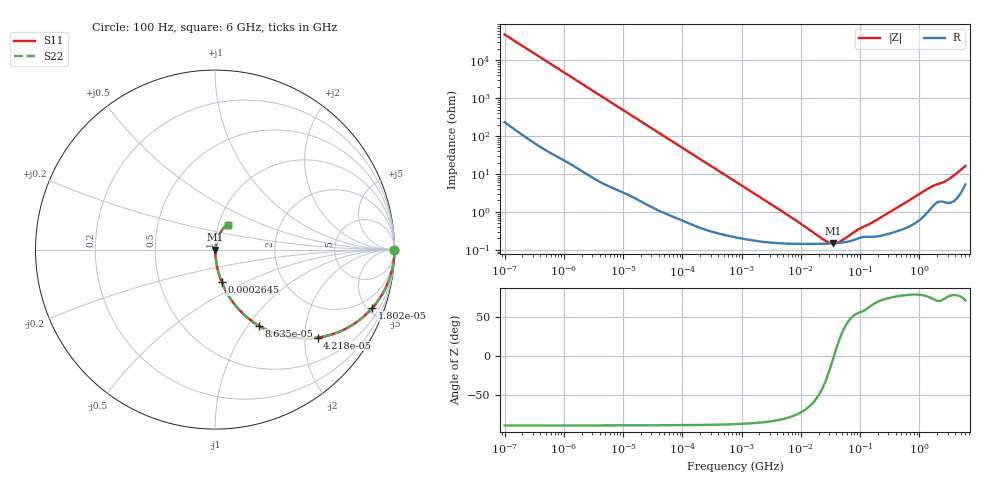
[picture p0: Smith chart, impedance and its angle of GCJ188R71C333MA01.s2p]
!Murata Part Number: GCJ188R71C333MA01
!These Parameters are Measured in Series Mode Connection
!Data Generated on Mar 13, 2026
!  o--ll--o
!Port1  Port2
!  o------o
!Operation Temp=25[degC], DC Bias Voltage=0[V]
!Freq. Start=100[Hz] Stop=6[GHz] 401[Steps]
# Hz S RI R 50
!Freq.(Hz) S11(Real) S11(Imag) S21(Real) S21(Imag) S12(Real) S12(Imag) S22(Real) S22(Imag)
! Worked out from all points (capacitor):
!   401 points, 100 Hz to 6 GHz, reference 50 ohm
!   read as one part in series: C = 33.2 nF near 109 Hz
!   lowest |Z| = 148 mohm at 34.83 MHz (marker M1)
!   series resonance near 36.44 MHz, so ESL is about 570 pH
!   S11 on the Smith chart (normalised r, x): 100 Hz: open; 18.02 kHz: 1.04, -5.40; 42.18 kHz: 1.02, -2.31; 86.35 kHz: 1.01, -1.13; 264.5 kHz: 1.01, -0.37; 6 GHz: 1.11, +0.31
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100  1 -0.00209  1.45e-05 0.00209  1.45e-05 0.00209  1 -0.00209
2008  0.9981 -0.0415  0.00194 0.0415  0.00194 0.0415  0.9981 -0.0415
6728  0.9803 -0.1362  0.0197 0.1362  0.0197 0.1362  0.9803 -0.1362
18016  0.8773 -0.3242  0.1227 0.3242  0.1227 0.3242  0.8773 -0.3242
26957  0.7636 -0.4208  0.2364 0.4208  0.2364 0.4208  0.7636 -0.4208
40335  0.5932 -0.4868  0.4068 0.4868  0.4068 0.4868  0.5932 -0.4868
42182  0.5717 -0.4904  0.4283 0.4904  0.4283 0.4904  0.5717 -0.4904
60352  0.3971 -0.4843  0.6029 0.4843  0.6029 0.4843  0.3971 -0.4843
86348  0.2459 -0.425  0.7541 0.425  0.7541 0.425  0.2459 -0.425
141303  0.1111 -0.3076  0.8889 0.3076  0.8889 0.3076  0.1111 -0.3076
264476  0.0365 -0.1791  0.9635 0.1791  0.9635 0.1791  0.0365 -0.1791
774597  0.00621 -0.0636  0.9938 0.0636  0.9938 0.0636  0.00621 -0.0636
1.555665e7  0.00144 -0.00265  0.9986 0.00265  0.9986 0.00265  0.00144 -0.00265
2.662322e7  0.00145 -0.000881  0.9986 0.000881  0.9986 0.000881  0.00145 -0.000881
3.482834e7  0.00147 -0.000125  0.9985 0.000125  0.9985 0.000125  0.00147 -0.000125
4.764863e7  0.00153 0.000748  0.9985 -0.000748  0.9985 -0.000748  0.00153 0.000748
9.326766e7  0.00199 0.00282  0.998 -0.00282  0.998 -0.00282  0.00199 0.00282
1.526266e8  0.00221 0.00449  0.9978 -0.00449  0.9978 -0.00449  0.00221 0.00449
3.124326e8  0.00276 0.00937  0.9972 -0.00937  0.9972 -0.00937  0.00276 0.00937
1.497423e9  0.0129 0.0411  0.9871 -0.0411  0.9871 -0.0411  0.0129 0.0411
2.931063e9  0.0211 0.063  0.9789 -0.063  0.9789 -0.063  0.0211 0.063
6e9  0.0698 0.1351  0.9302 -0.1351  0.9302 -0.1351  0.0698 0.1351
